// TwinCAT 3 PLC project recipetest
// ProgramVersion: 3.1.4022.7
// libraries:
//   Recipe Management, * (System)
//   Tc2_Standard, * (Beckhoff Automation GmbH)
//   Tc2_System, * (Beckhoff Automation GmbH)
//   Tc3_Module, * (Beckhoff Automation GmbH)
//   VisuDialogs, * (System)
//   VisuSymbols,3.5.10.0,System
// project tree:
//   / GlobalTextList.TcGTLO, PlcTask.TcTTO, RecipeManager.TcRMO, Visualization Manager.TcVMO
//   GVLs/ GVL_recipe.TcGVL
//   POUs/ MAIN.TcPOU
//   VISUs/ recipe_save_and_load.TcVIS
// real-time tasks:
//   TASK PlcTask: cycle T#10ms, priority 20, ADS port 350

CONFIGURATION recipetest
    RESOURCE PLC ON TwinCAT3
        TASK PlcTask(INTERVAL := T#10ms, PRIORITY := 20);
        PROGRAM MAIN WITH PlcTask : MAIN;
    END_RESOURCE
END_CONFIGURATION

// ---- GVLs/GVL_recipe.TcGVL
VAR_GLOBAL
	velocity:LREAL;
	distance:LREAL;
	version:STRING;
	number:INT;
	boxL:LREAL;
	boxW:LREAL;
	boxH:LREAL;
END_VAR

// ---- POUs/MAIN.TcPOU
PROGRAM MAIN
VAR
	fb_recipemancommands:recipemancommands;//配方功能块
	f_trig_save,f_trig_load:f_trig;//用于触发保存/读取的下降沿功能块
	bsave,bload:BOOL;//保存，读取按钮
	recipedefinitionname:STRING:='BOX';//配方表名称
	sfilepath:STRING:='E:\recipefiles\box';//文件路径
	filename:STRING:='box1';//文件名
END_VAR

f_trig_save(CLK:= bsave, Q=> );
f_trig_load(CLK:= bload, Q=> );

IF f_trig_save.Q THEN
	fb_recipemancommands.CreateRecipe(RecipeDefinitionName:= recipedefinitionname, RecipeName:= 'parameter1');
	fb_recipemancommands.ReadAndSaveRecipeAs(RecipeDefinitionName:= recipedefinitionname, RecipeName:= 'parameter1',
	FileName:= concat(concat(concat(sfilepath,'\'),filename),'.txtrecipe'));
END_IF

IF f_trig_load.Q THEN
	fb_recipemancommands.CreateRecipe(RecipeDefinitionName:= recipedefinitionname, RecipeName:= 'parameter1');
	fb_recipemancommands.LoadFromAndWriteRecipe(RecipeDefinitionName:= recipedefinitionname, RecipeName:= 'parameter1',
	FileName:= concat(concat(concat(sfilepath,'\'),filename),'.txtrecipe'));
END_IF

END_PROGRAM

// ---- GlobalTextList.TcGTLO
TEXTLIST GlobalTextList
  993 = 'boxH:'
  27 = 'boxH:%f'
  939 = 'boxH:%s'
  325 = 'boxL:'
  439 = 'boxL:%f'
  306 = 'boxL:%s'
  66 = 'boxW:'
  801 = 'boxW:%f'
  608 = 'boxW:%s'
  253 = 'distance'
  679 = 'distance:'
  226 = 'distance:%f'
  391 = 'number:'
  975 = 'number:%s'
  821 = 'Parameter Modification'
  832 = 'velocity:'
  266 = 'velocity:%f'
  231 = 'version:'
  737 = 'version:%s'
  183 = '保存配方'
  730 = '文件名:%s'
  519 = '文件路径:%s'
  224 = '读取配方'
  232 = '配方表名称:%s'
END_TEXTLIST

// ---- VISUs/recipe_save_and_load.TcVIS
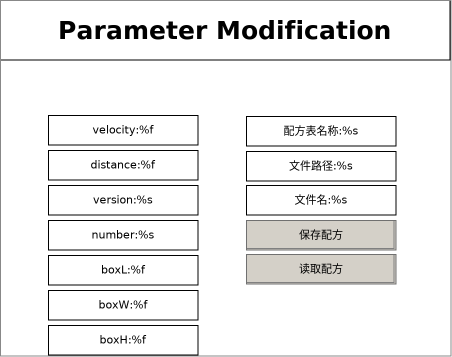
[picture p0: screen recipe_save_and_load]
VISUALIZATION recipe_save_and_load  // 452x357
    Rectangle (0,0 450x60), "Parameter Modification"
    Rectangle (48,115 150x30), "velocity:%f", text variable: velocity
        OnMouseClick: write velocity via Default
    Rectangle (48,150 150x30), "distance:%f", text variable: distance
        OnMouseClick: write the text variable via Default
    Rectangle (48,185 150x30), "version:%s", text variable: version
        OnMouseClick: write the text variable via Default
    Rectangle (48,220 150x30), "number:%s", text variable: number
        OnMouseClick: write the text variable via Default
    Rectangle (246,116 150x30), "配方表名称:%s", text variable: MAIN.recipedefinitionname
        OnMouseClick: write the text variable via Default
    Rectangle (48,255 150x30), "boxL:%f", text variable: boxL
        OnMouseClick: write the text variable via Default
    Rectangle (48,290 150x30), "boxW:%f", text variable: boxW
        OnMouseClick: write the text variable via Default
    Rectangle (48,325 150x30), "boxH:%f", text variable: boxH
        OnMouseClick: write the text variable via Default
    Rectangle (246,151 150x30), "文件路径:%s", text variable: MAIN.sfilepath
        OnMouseClick: write the text variable via Default
    Rectangle (246,185 150x30), "文件名:%s", text variable: MAIN.filename
        OnMouseClick: write the text variable via Default
    Button (246,220 150x30), "保存配方"
        tap MAIN.bsave
    Button (246,254 150x30), "读取配方"
        tap MAIN.bload
END_VISUALIZATION
